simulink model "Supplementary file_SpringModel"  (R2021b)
settings: Solver=VariableStepAuto  StartTime=0.0  StopTime=10.0  RelTol=1e-3
model workspace (MAT data in the model file):
  b = 0.001
  k = 0.023
  m = 0.002

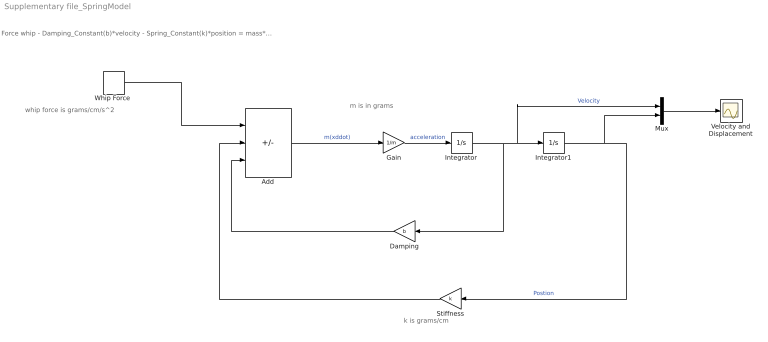
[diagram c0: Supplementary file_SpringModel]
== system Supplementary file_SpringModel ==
  note: whip force is grams/cm/s^2
  note: k is grams/cm
  note: m is in grams
  note: Force whip - Damping_Constant(b)*velocity - Spring_Constant(k)*position = mass*(acceleration)
  Add : Sum  Inputs=+--
  Damping : Gain  Gain=b
  Gain : Gain  Gain=1/m
  Integrator : Integrator
  Integrator1 : Integrator
  Mux : Mux  Inputs=2
  Stiffness : Gain  Gain=k
  Velocity and Displacement : Scope
  "Whip Force " : DiscretePulseGenerator  PulseType=Time based  Amplitude=0.26  Period=10
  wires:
  Add/1 -> Gain/1  "m(xddot)"
  Gain/1 -> Integrator/1  "acceleration"
  Integrator/1 -> Damping/1, Mux/1, Integrator1/1  "Velocity"
  Damping/1 -> Add/3
  Stiffness/1 -> Add/2
  Integrator1/1 -> Stiffness/1, Mux/2  "Postion"
  Mux/1 -> Velocity and Displacement/1
  "Whip Force "/1 -> Add/1
